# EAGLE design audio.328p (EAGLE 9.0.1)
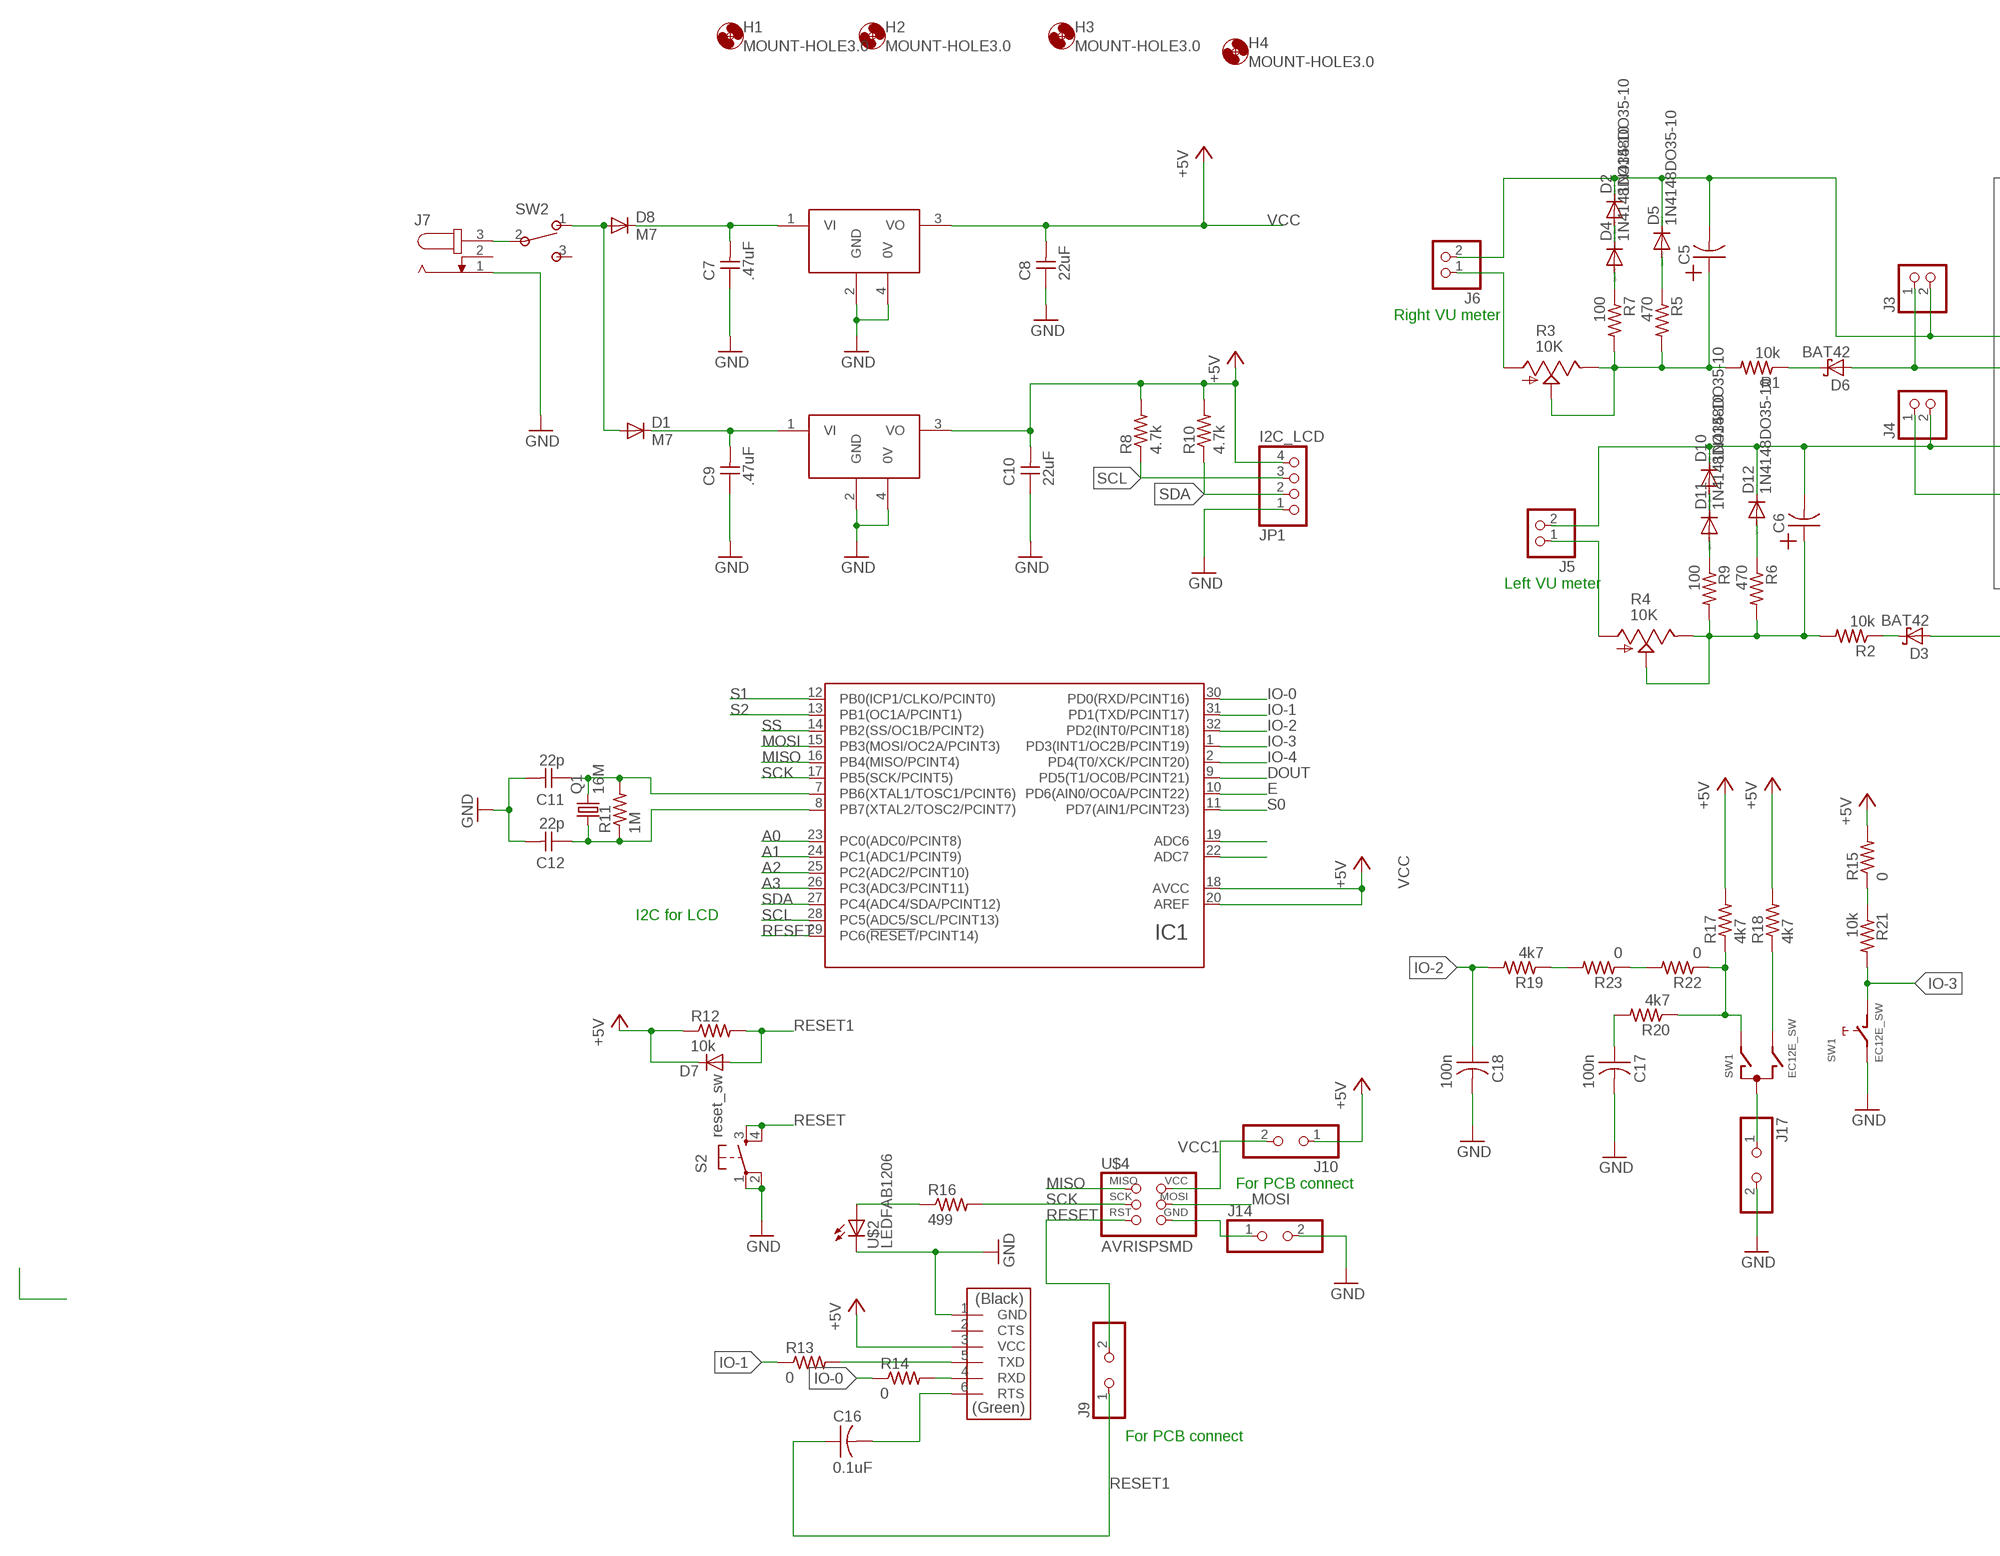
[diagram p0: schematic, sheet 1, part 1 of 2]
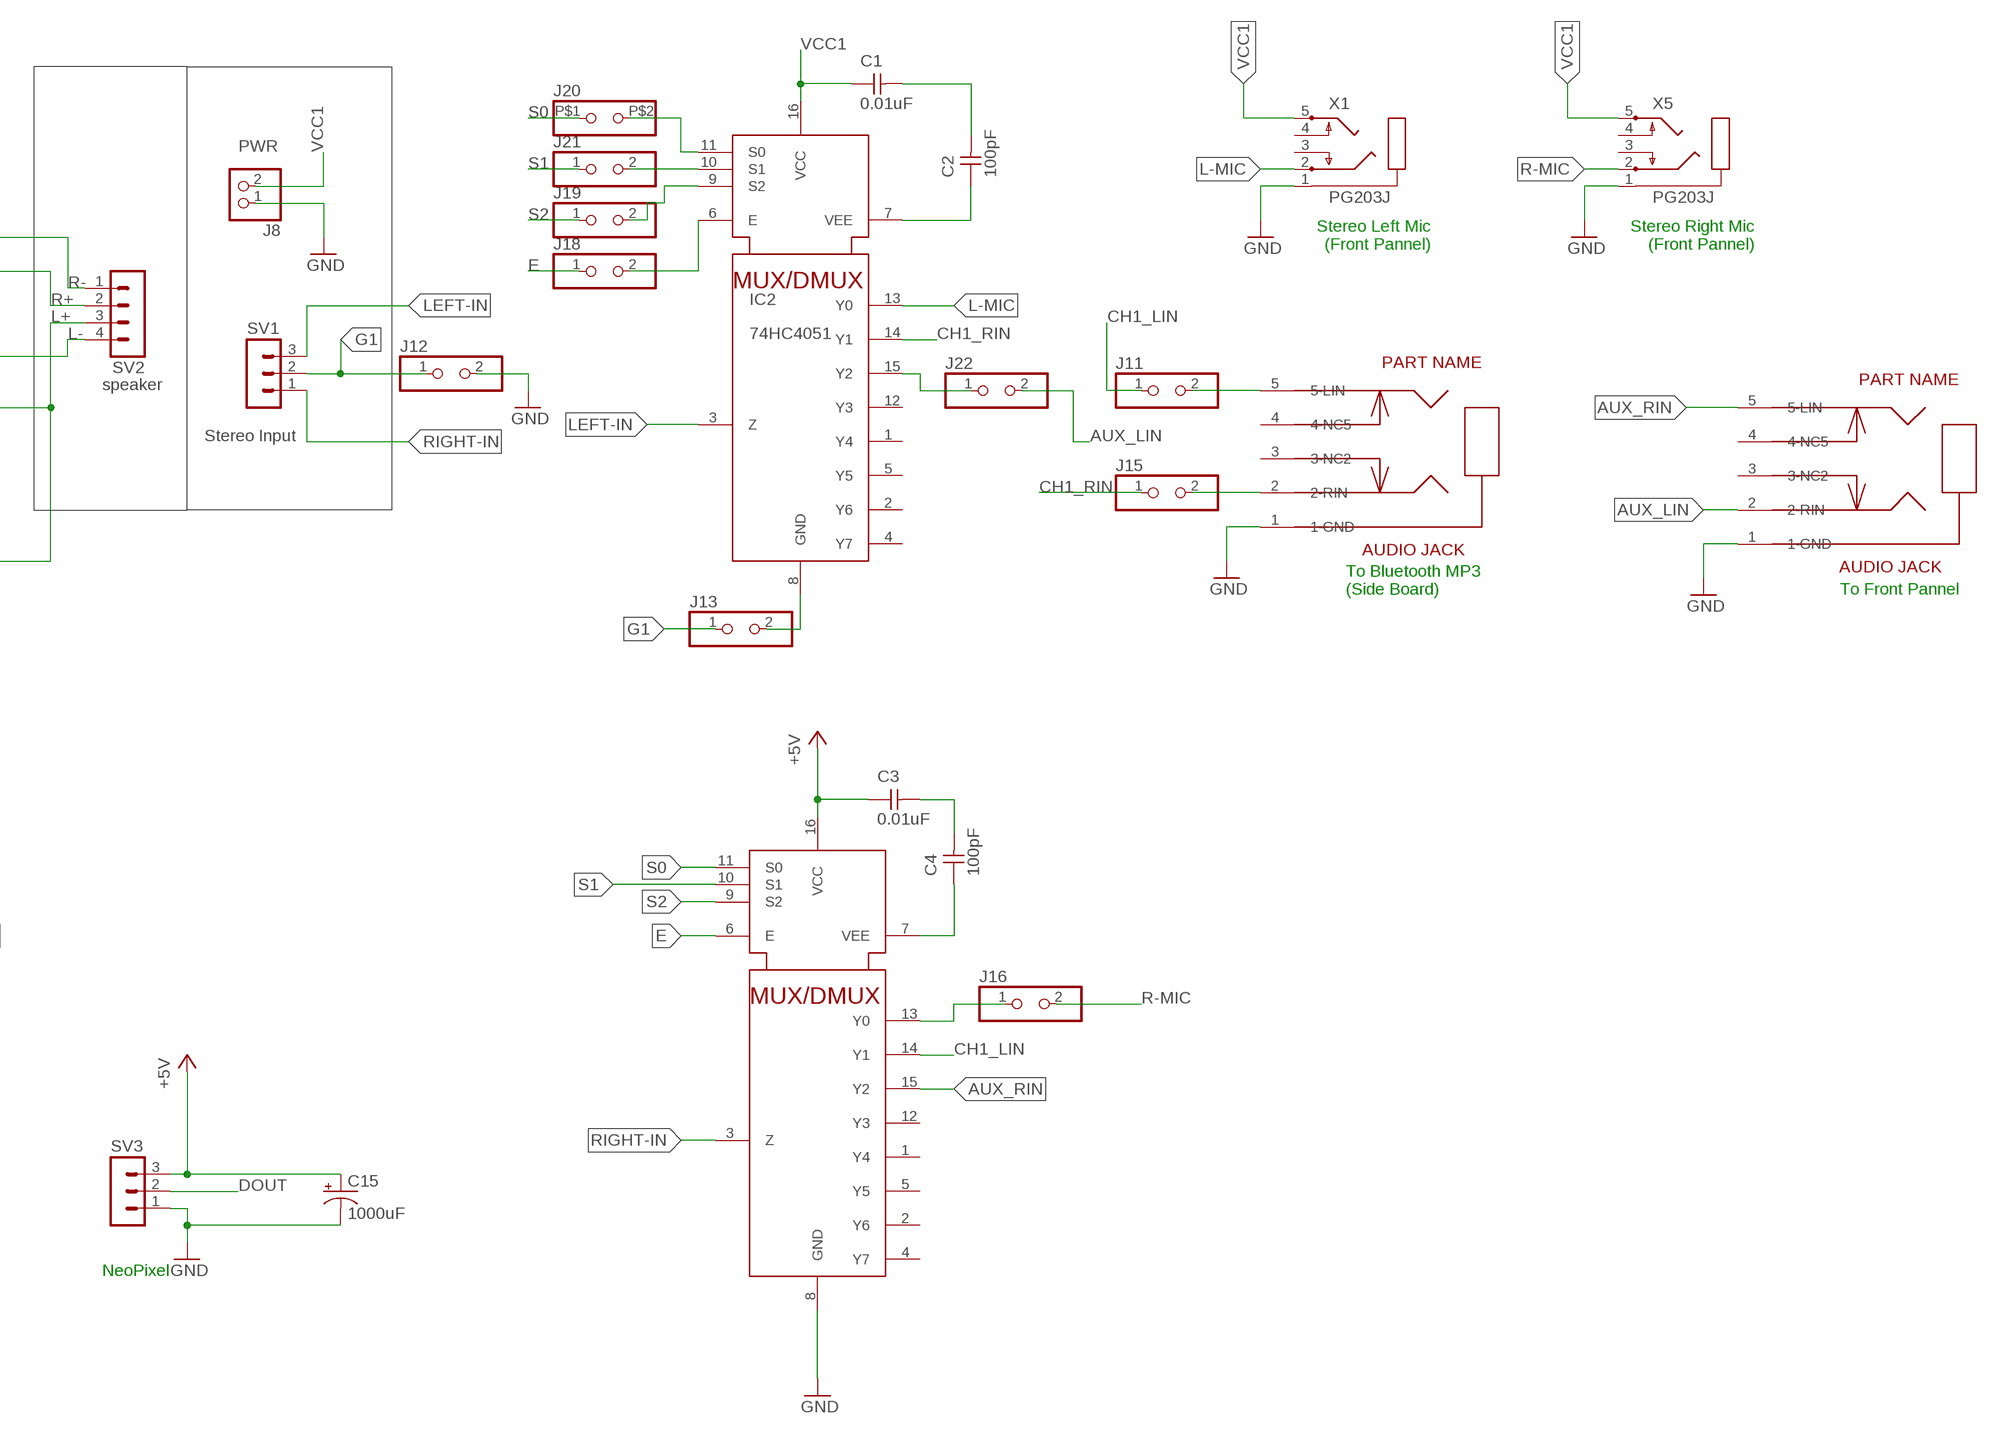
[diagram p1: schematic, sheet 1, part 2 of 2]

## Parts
C1  0.01uF  CAP-UNPOLARIZEDFAB  [C1206FAB]
C2  100pF  CAP-UNPOLARIZEDFAB  [C1206FAB]
C3  0.01uF  CAP-UNPOLARIZEDFAB  [C1206FAB]
C4  100pF  CAP-UNPOLARIZEDFAB  [C1206FAB]
C5  CAP_POL5MM  [5X11MMCAP]
C6  CAP_POL5MM  [5X11MMCAP]
C7  .47uF  CAP-UNPOLARIZEDFAB  [C1206FAB]
C8  22uF  CAP-UNPOLARIZEDFAB  [C1206FAB]
C9  .47uF  CAP-UNPOLARIZEDFAB  [C1206FAB]
C10  22uF  CAP-UNPOLARIZEDFAB  [C1206FAB]
C11  22p  CAP-UNPOLARIZEDFAB  [C1206FAB]
C12  22p  CAP-UNPOLARIZEDFAB  [C1206FAB]
C15  1000uF  CPOL-USE5-10.5  [E5-10,5]
C16  0.1uF  CAP-US1206FAB  [C1206FAB]
C17  100n  CAP-US1206FAB  [C1206FAB]
C18  100n  CAP-US1206FAB  [C1206FAB]
D1  M7  DIODESOD123  [SOD123]
D2  1N4148DO35-10  [DO35-10]
D3  BAT42  [DO35-10]
D4  1N4148DO35-10  [DO35-10]
D5  1N4148DO35-10  [DO35-10]
D6  BAT42  [DO35-10]
D7  DIODESOD123  [SOD123]
D8  M7  DIODESOD123  [SOD123]
D10  1N4148DO35-10  [DO35-10]
D11  1N4148DO35-10  [DO35-10]
D12  1N4148DO35-10  [DO35-10]
H1  MOUNT-HOLE3.0  [3,0]
H2  MOUNT-HOLE3.0  [3,0]
H3  MOUNT-HOLE3.0  [3,0]
H4  MOUNT-HOLE3.0  [3,0]
IC1  ATMEGA48/88/168/328-AU  [TQFP32-08]
IC2  74HC4051  [D_R-PDSO-G16]
IC3  74HC4051  [D_R-PDSO-G16]
J1  BLUE TOOTH  PJ307L  [PJ307L]
J2  PJ307L  [PJ307L]
J3  5267-2P  [MOLEX5267-2P]
J4  5267-2P  [MOLEX5267-2P]
J5  5267-2P  [MOLEX5267-2P]
J6  5267-2P  [MOLEX5267-2P]
J7  JACK-PLUG1  [SPC4078]
J8  5267-2P  [MOLEX5267-2P]
J9  JMPPER18MM  [1X2PJMP18MM]
J10  JMPPER18MM  [1X2PJMP18MM]
J11  JMPPER5M8  [1X2PJMP5M8]
J12  JMPPER5M8  [1X2PJMP5M8]
J13  JMPPER5M8  [1X2PJMP5M8]
J14  JMPPER5M8  [1X2PJMP5M8]
J15  JMPPER5M8  [1X2PJMP5M8]
J16  JMPPER5M8  [1X2PJMP5M8]
J17  JMPPER5M8  [1X2PJMP5M8]
J18  JMPPER5M8  [1X2PJMP5M8]
J19  JMPPER5M8  [1X2PJMP5M8]
J20  JMPPER12MM  [1X2PJMP12MM]
J21  JMPPER5M8  [1X2PJMP5M8]
J22  JMPPER5M8  [1X2PJMP5M8]
JP1  I2C_LCD  PINHD-1X4  [1X04]
M1  FTDI-THT-HEADER  [1X06]
Q1  16M  CRYSTALSM49  [SM49]
R1  10k  RES-US1206FAB  [R1206FAB]
R2  10k  RES-US1206FAB  [R1206FAB]
R3  10K  POT1K_ANGLE  [EVUFXK]
R4  10K  POT1K_ANGLE  [EVUFXK]
R5  470  RES-US1206FAB  [R1206FAB]
R6  470  RES-US1206FAB  [R1206FAB]
R7  100  RES-US1206FAB  [R1206FAB]
R8  4.7k  RES-US1206FAB  [R1206FAB]
R9  100  RES-US1206FAB  [R1206FAB]
R10  4.7k  RES-US1206FAB  [R1206FAB]
R11  1M  RES-US1206FAB  [R1206FAB]
R12  10k  RES-US1206FAB  [R1206FAB]
R13  0  RES-US1206FAB  [R1206FAB]
R14  0  RES-US1206FAB  [R1206FAB]
R15  0  RES-US1206FAB  [R1206FAB]
R16  499  RES-US1206FAB  [R1206FAB]
R17  4k7  RES-US1206FAB  [R1206FAB]
R18  4k7  RES-US1206FAB  [R1206FAB]
R19  4k7  RES-US1206FAB  [R1206FAB]
R20  4k7  RES-US1206FAB  [R1206FAB]
R21  10k  RES-US1206FAB  [R1206FAB]
R22  0  RES-US1206FAB  [R1206FAB]
R23  0  RES-US1206FAB  [R1206FAB]
S2  reset_sw  6MM_SWITCH6MM_SWITCH  [6MM_SWITCH]
SV1  MA03-1  [MA03-1]
SV2  MA04-1  [MA04-1]
SV3  MA03-1  [MA03-1]
SW1  EC12E_SW  [ALPS_EC12E_SW]
SW2  SLIDE-3PSW  [3P5_08]
U1  LM2940-5  LM2940  [SOT223]
U2  LM2940  [SOT223]
U$2  LEDFAB1206  [LED1206FAB]
U$4  AVRISPSMD  [2X03SMD]
X1  PG203J  [PG203J]
X5  PG203J  [PG203J]

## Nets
+5V: C3.1 C10.2 C15.+ D7.CATHODE(C) IC3.16(VCC) J10.1 JP1.4 M1.3(VCC) R8.2 R10.2 R12.1 R15.2 R17.2 R18.2 SV3.3 U2.3(VO)
A0: IC1.23(PC0(ADC0/PCINT8))
A1: IC1.24(PC1(ADC1/PCINT9))
A2: IC1.25(PC2(ADC2/PCINT10))
A3: IC1.26(PC3(ADC3/PCINT11))
AUX_LIN: J2.2(2-RIN) J22.2
AUX_RIN: IC3.15(Y2) J2.5(5-LIN)
CH1_LIN: IC3.14(Y1) J11.1
CH1_RIN: IC2.14(Y1) J15.1
DOUT: IC1.9(PD5(T1/OC0B/PCINT21)) SV3.2
E: IC1.10(PD6(AIN0/OC0A/PCINT22)) IC3.6(E) J18.1
G1: J12.1 J13.1 SV1.2
GND: C7.1 C8.1 C9.1 C10.1 C11.2 C12.2 C15.- C17.2 C18.2 IC3.8(GND) J1.1(1-GND) J2.1(1-GND) J7.1 J8.1 J12.2 J14.2 J17.2 JP1.1 M1.1(GND) S2.1(P) S2.2(P1) SV3.1 SW1.E U1.2(GND) U1.4(0V) U2.2(GND) U2.4(0V) U$2.2(C) X1.1 X5.1
IO-0: IC1.30(PD0(RXD/PCINT16)) R14.1
IO-1: IC1.31(PD1(TXD/PCINT17)) R13.1
IO-2: C18.1 IC1.32(PD2(INT0/PCINT18)) R19.2
IO-3: IC1.1(PD3(INT1/OC2B/PCINT19)) R21.2 SW1.D
IO-4: IC1.2(PD4(T0/XCK/PCINT20))
L+: D3.A J4.1 SV2.3
L-: C6.P$2(M) D10.C D12.C J4.2 J5.2 SV2.4
L-MIC: IC2.13(Y0) X1.2
LEFT-IN: IC2.3(Z) SV1.3
MISO: IC1.16(PB4(MISO/PCINT4)) U$4.1(MISO)
MOSI: IC1.15(PB3(MOSI/OC2A/PCINT3)) U$4.4(MOSI)
N$1: C1.2 C2.2
N$2: C2.1 IC2.7(VEE)
N$3: C3.2 C4.2
N$4: C4.1 IC3.7(VEE)
N$5: J7.3 SW2.2
N$6: C7.2 D8.CATHODE(C) U1.1(VI)
N$8: IC1.19(ADC6)
N$9: D11.A R9.1
N$10: D12.A R6.1
N$11: D10.A D11.C
N$12: D6.C R1.1
N$13: C6.P$1(P) R2.2 R4.2(S) R4.3(E) R6.2 R9.2
N$14: J5.1 R4.1(A)
N$15: C9.2 D1.CATHODE(C) U2.1(VI)
N$16: C5.P$1(P) R1.2 R3.2(S) R3.3(E) R5.2 R7.2
N$18: D4.A R7.1
N$19: D5.A R5.1
N$20: D2.A D4.C
N$21: J6.1 R3.1(A)
N$22: IC1.22(ADC7)
N$26: C11.1 IC1.7(PB6(XTAL1/TOSC1/PCINT6)) Q1.2 R11.2
N$27: C12.1 IC1.8(PB7(XTAL2/TOSC2/PCINT7)) Q1.1 R11.1
N$28: R16.1 U$2.1(A)
N$29: R18.1 SW1.B
N$30: C16.2 M1.6(RTS)
N$31: R17.1 R20.1 R22.1 SW1.A
N$32: C17.1 R20.2
N$33: D1.ANODE(A) D8.ANODE(A) SW2.1
N$34: M1.4(RXD) R14.2
N$35: M1.5(TXD) R13.2
N$36: R15.1 R21.1
N$37: R19.1 R23.2
N$38: R22.2 R23.1
N$39: J1.2(2-RIN) J15.2
N$40: J14.1 U$4.6(GND)
N$41: IC2.8(GND) J13.2
N$42: J1.5(5-LIN) J11.2
N$43: J17.1 SW1.C
N$44: IC3.13(Y0) J16.1
N$45: IC2.10(S1) J21.2
N$46: IC2.11(S0) J20.P$2
N$47: IC2.9(S2) J19.2
N$48: IC2.6(E) J18.2
N$49: IC2.15(Y2) J22.1
N$50: D3.C R2.1
R+: D6.A J3.1 SV2.2
R-: C5.P$2(M) D2.C D5.C J3.2 J6.2 SV2.1
R-MIC: J16.2 X5.2
RESET: IC1.29(PC6(!RESET!/PCINT14)) J9.2 S2.3(S) S2.4(S1) U$4.5(RST)
RESET1: C16.1 D7.ANODE(A) J9.1 R12.2
RIGHT-IN: IC3.3(Z) SV1.1
S0: IC1.11(PD7(AIN1/PCINT23)) IC3.11(S0) J20.P$1
S1: IC1.12(PB0(ICP1/CLKO/PCINT0)) IC3.10(S1) J21.1
S2: IC1.13(PB1(OC1A/PCINT1)) IC3.9(S2) J19.1
SCK: IC1.17(PB5(SCK/PCINT5)) R16.2 U$4.3(SCK)
SCL: IC1.28(PC5(ADC5/SCL/PCINT13)) JP1.3 R8.1
SDA: IC1.27(PC4(ADC4/SDA/PCINT12)) JP1.2 R10.1
SS: IC1.14(PB2(SS/OC1B/PCINT2))
VCC: C8.2 IC1.18(AVCC) IC1.20(AREF) U1.3(VO) ; supply symbol labelled +5V
VCC1: C1.1 IC2.16(VCC) J8.2 J10.2 U$4.2(VCC) X1.5 X5.5
Unconnected: IC2.1(Y4) IC2.2(Y6) IC2.4(Y7) IC2.5(Y5) IC2.12(Y3) IC3.1(Y4) IC3.2(Y6) IC3.4(Y7) IC3.5(Y5) IC3.12(Y3) J1.3(3-NC2) J1.4(4-NC5) J2.3(3-NC2) J2.4(4-NC5) J7.2 M1.2(CTS) SW1.GND1(G) SW1.GND2(G) SW2.3 X1.3 X1.4 X5.3 X5.4

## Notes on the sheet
- PWR
- Right VU meter
- Stereo Left Mic
  (Front Pannel)
- Stereo Right Mic
  (Front Pannel)
- speaker
- Stereo Input
- Left VU meter
- To Bluetooth MP3
  (Side Board)
- To Front Pannel
- I2C for LCD
- For PCB connect
- NeoPixel
- For PCB connect

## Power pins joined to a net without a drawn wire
GND: IC1.3(GND) IC1.5(GND) IC1.21(GND)
VCC: IC1.4(VCC) IC1.6(VCC)

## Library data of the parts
C1-C4 C7-C12 = fab:CAP-UNPOLARIZED
C5 C6 = discrete_ys:CAP_POL5MM
C15 = rcl:CPOL-US: POLARIZED CAPACITOR, American symbol; SPICEPREFIX: C
C16-C18 = fab:CAP-US
D1 D7 D8 = fab:DIODE: DIODE
D2 D4 D5 D10-D12 = diode:1N4148: DIODE
D3 D6 = diode:BAT42: DIODE
H1-H4 = holes:MOUNT-HOLE: MOUNTING HOLE with drill center marker
IC1 = atmel_tiny24-44-84tiny48-88mega48-88-168-328:ATMEGA48/88/168/328
IC2 IC3 = audio_basic:74HC4051
J1 J2 = audio_basic:PJ307L
J3-J6 J8 = connector_ys:5267-2P
J7 = con-jack:JACK-PLUG: DC POWER JACK Power Jack, DC, Right Angle, Through Hole, Rated 5A at 16VDC, PC Terminals Distributor: Farnell (www.Farnell.de) Drawing: 84N1161.pdf / 84N1162.pdf Manufacturer: SPC Technology (www.spctechnology.com) Type: SPC4077 / SPC 4078; OC_FARNELL: unknown; OC_NEWARK: unknown
J9 J10 = discrete_ys:JMPPER18MM
J11-J19 J21 J22 = discrete_ys:JMPPER5M8
J20 = discrete_ys:JMPPER12MM
JP1 = pinhead:PINHD-1X4: PIN HEADER
M1 = fab:FTDI-THT-HEADER
Q1 = crystal:CRYSTAL: CRYSTAL; OC_FARNELL: unknown; OC_NEWARK: unknown
R1 R2 R5-R23 = fab:RES-US: Resistor (US Symbol)
R3 R4 = discrete_ys:POT1K_ANGLE
S2 = fab:6MM_SWITCH: OMRON SWITCH
SV1 SV3 = con-lstb:MA03-1: PIN HEADER; OC_FARNELL: unknown; OC_NEWARK: unknown
SV2 = con-lstb:MA04-1: PIN HEADER; OC_FARNELL: unknown; OC_NEWARK: unknown
SW1 = switch-alps:EC12E_SW: ALPS rotary Encoder EC12E series with switch; MPN: EC12E2424407; OC_FARNELL: 1520813; OC_NEWARK: 74M1068
SW2 = connector_ys:SLIDE-3PSW
U1 U2 = discrete_ys:LM2940
U$2 = fab:LED: LED
U$4 = fab:AVRISP
X1 X5 = con-hirschmann:PG203J: MIC/HEADPHONE JACK KS-S stereo microphone/headphone jack PG203JN (Schukat); OC_FARNELL: unknown; OC_NEWARK: unknown

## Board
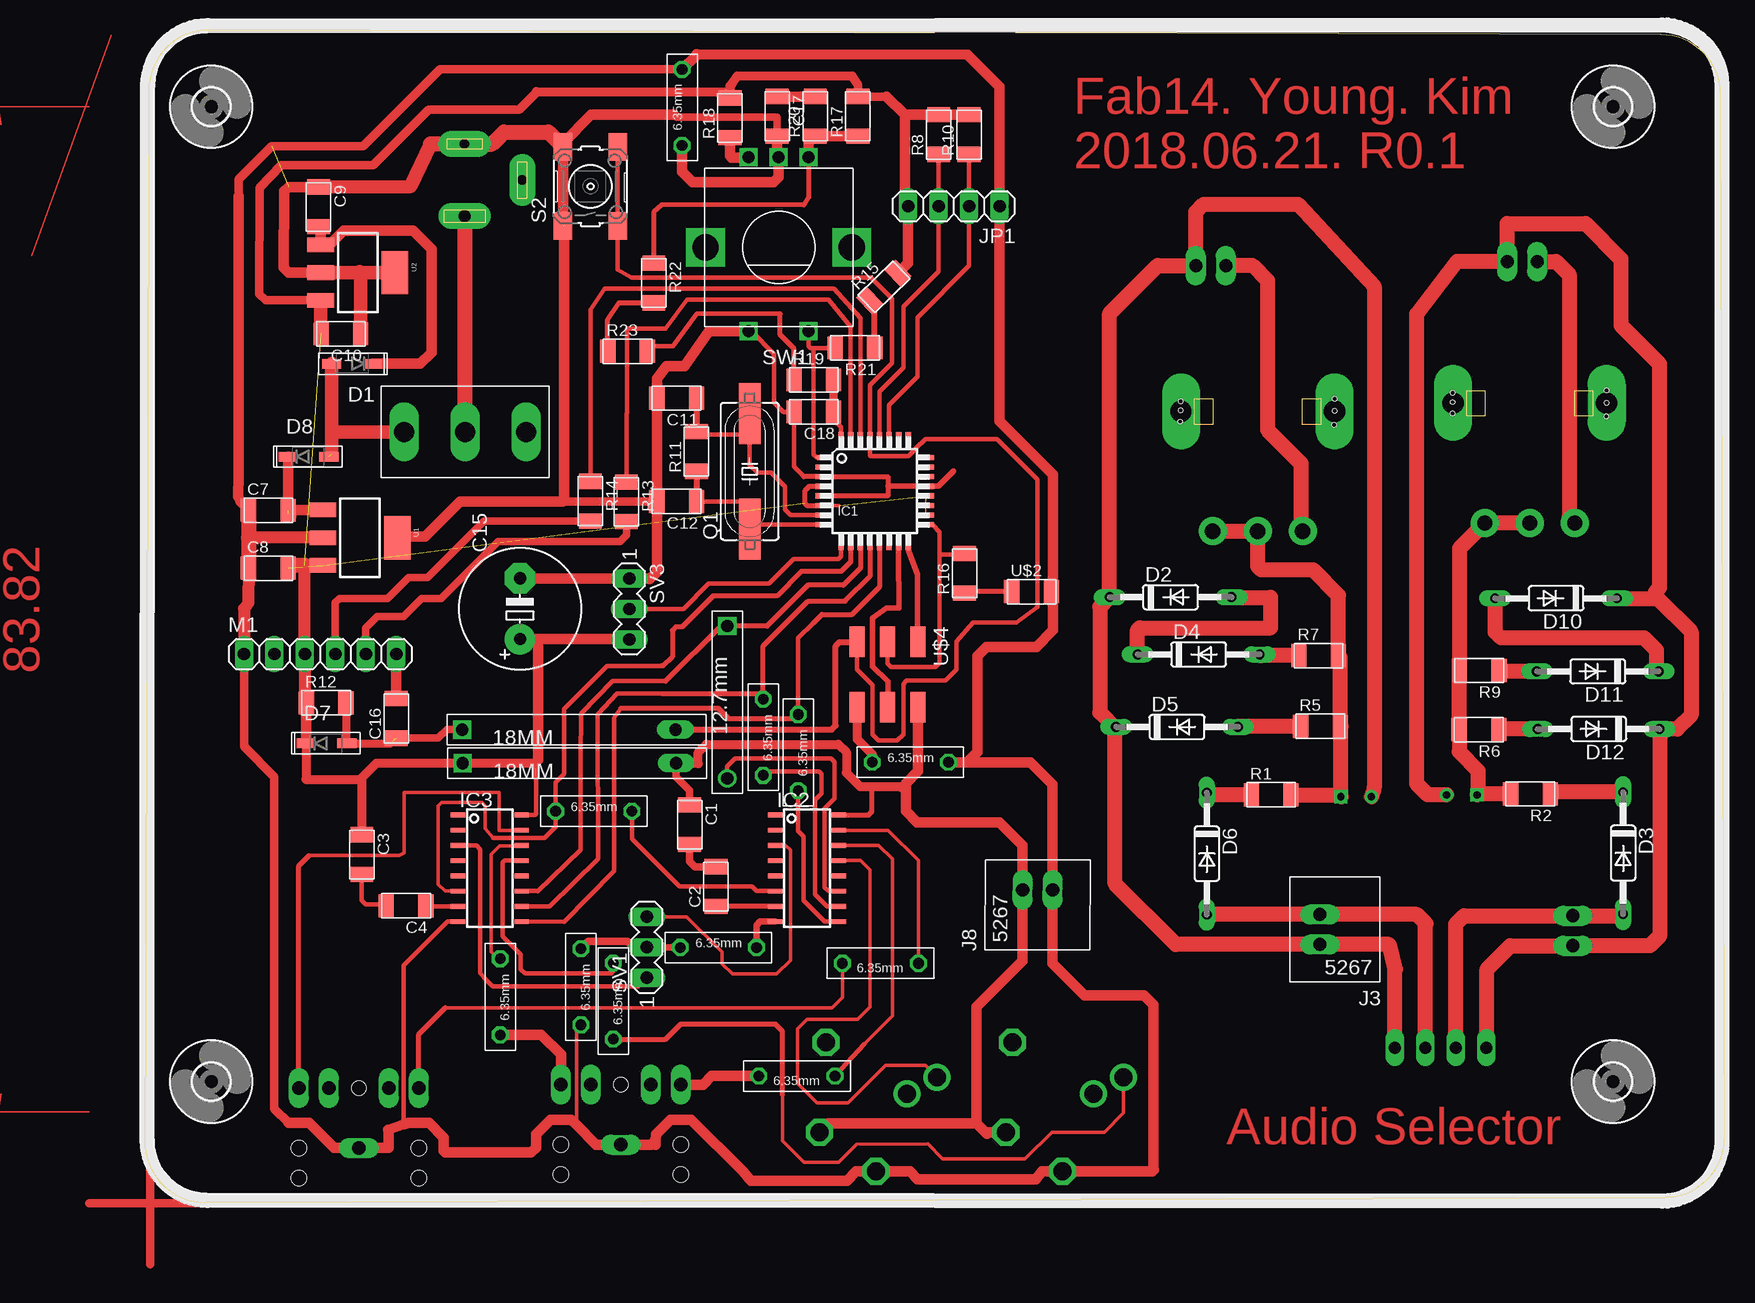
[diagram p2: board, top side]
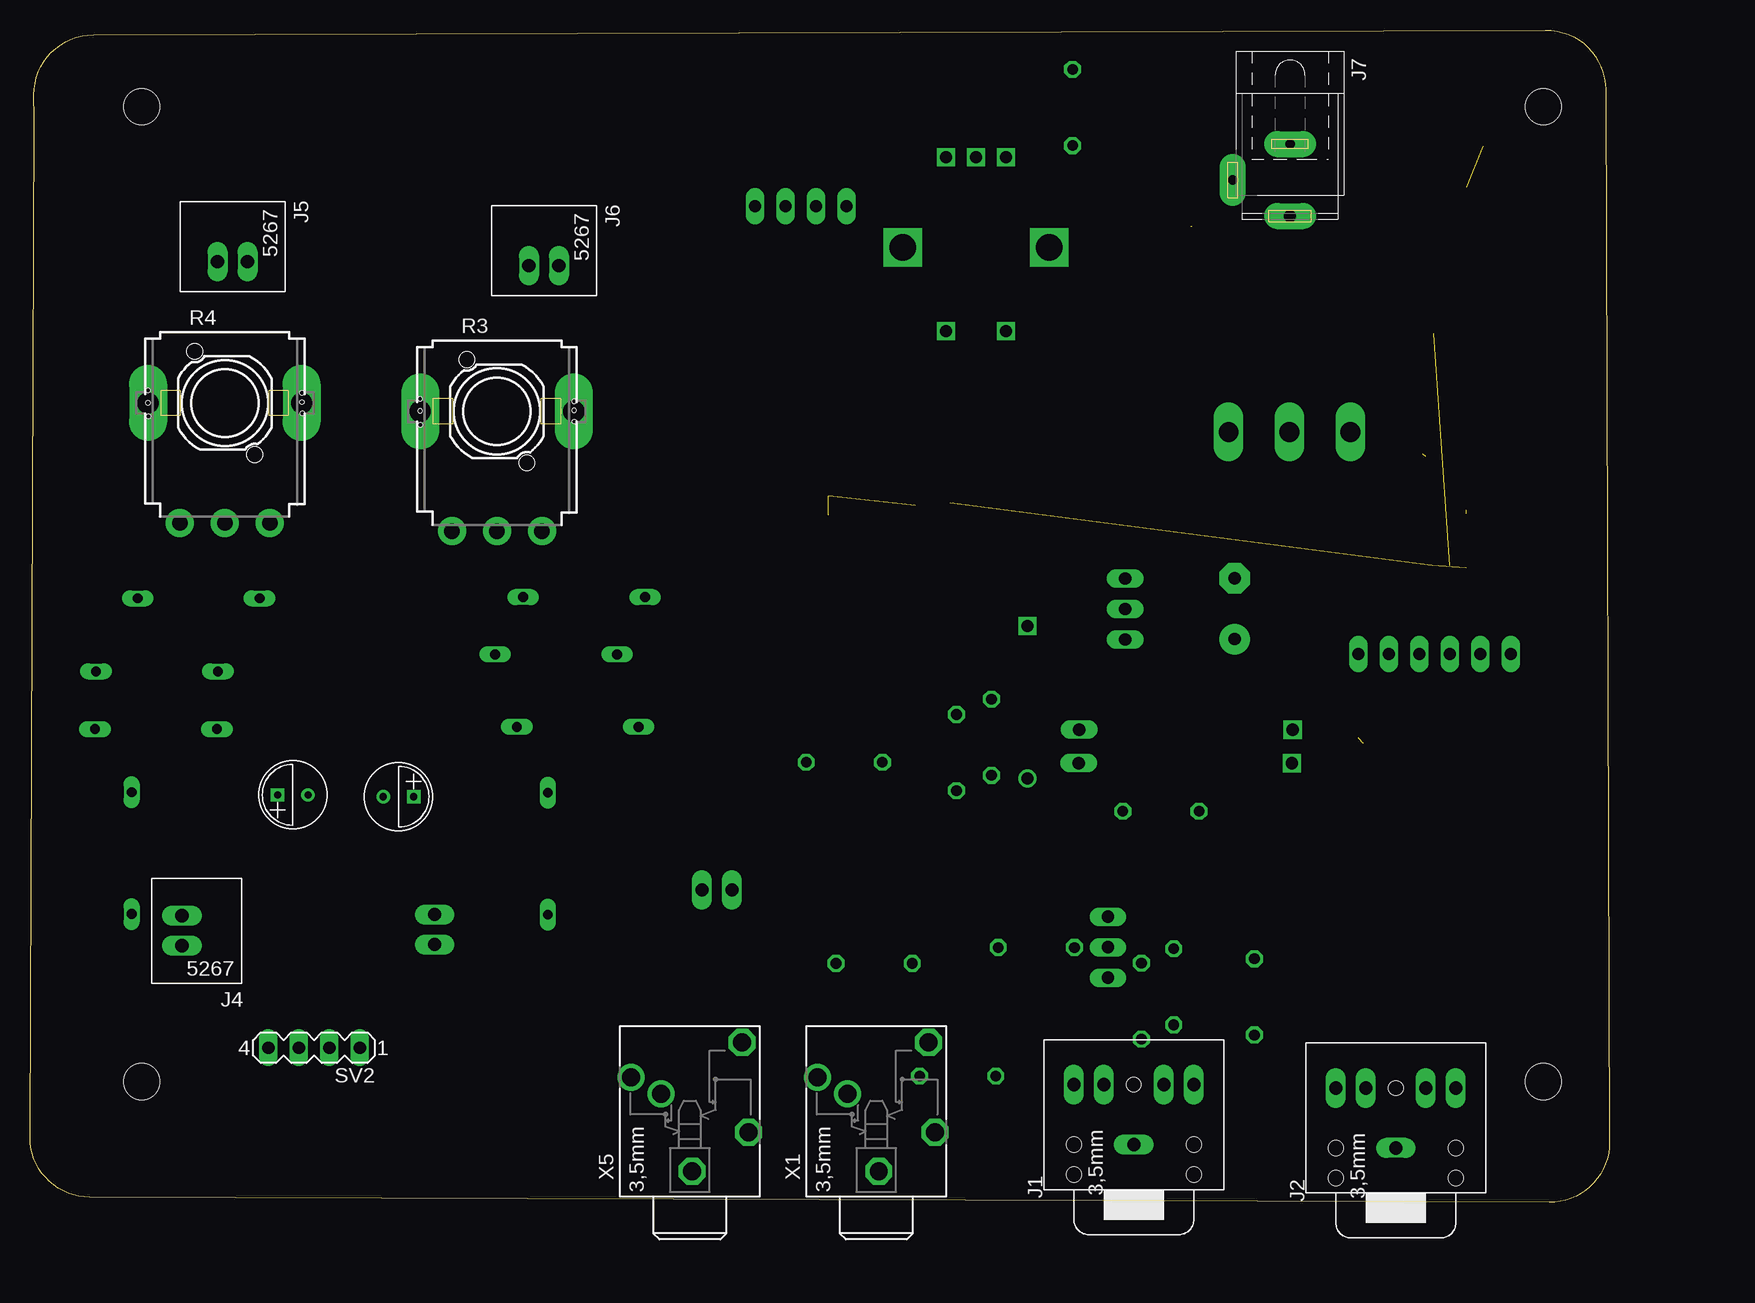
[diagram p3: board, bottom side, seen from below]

Size 131.67 x 97.73 mm. Coordinates in mm from the lower left corner, seen from the top.
Outline: 131.33,90.36 131.34,92.32 arc90 126.35,97.33 5.34,97.73 arc90 0.32,92.75 0,5.02 arc90 5.02,0 126.68,0.42 arc90 131.67,5.44 131.33,90.36
Copper layers (1*16): Top 0.035mm / dielectric 1.5mm / Bottom 0.035mm
Design rules "default *": minimum track width 6mil, minimum drill 0.35mm, track to track 6mil, track to pad 1mil, pad to pad 6mil, via to via 6mil, smd to smd 6mil, copper to edge 40mil, drill to drill 6mil, minimum pad ring 10mil, minimum via ring 8mil, stop-mask expansion 4mil, vias tented up to drill 0mil, thermal gap 10mil

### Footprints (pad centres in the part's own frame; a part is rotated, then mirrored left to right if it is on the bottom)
C1206FAB = smd 1.27 x 1.905: 1 -1.651,0; 2 1.651,0
5X11MMCAP = drill 0.6 square: P$1 0,1.27 | drill 0.6: P$2 0,-1.27
E5-10,5 = drill 1.016 pad 2.54: + -2.54,0 | drill 1.016 pad 2.54 octagon: - 2.54,0
SOD123 = smd 1.6 x 0.8: ANODE 1.7,0; CATHODE -1.7,0
DO35-10 = drill 0.813 long: A 5.08,0; C -5.08,0
3,0 = hole 3: 0,0
TQFP32-08 = smd 1.27 x 0.457: 1 -4.293,2.8 | smd 1.27 x 0.432: 2 -4.293,2; 3 -4.293,1.2; 4 -4.293,0.4; 5 -4.293,-0.4; 6 -4.293,-1.2; 7 -4.293,-2; 8 -4.293,-2.8; 17 4.293,-2.8; 18 4.293,-2; 19 4.293,-1.2; 20 4.293,-0.4; 21 4.293,0.4; 22 4.293,1.2; 23 4.293,2; 24 4.293,2.8 | smd 0.432 x 1.27: 9 -2.8,-4.293; 10 -2,-4.293; 11 -1.2,-4.293; 12 -0.4,-4.293; 13 0.4,-4.293; 14 1.2,-4.293; 15 2,-4.293; 16 2.8,-4.293; 25 2.8,4.293; 26 2,4.293; 27 1.2,4.293; 28 0.4,4.293; 29 -0.4,4.293; 30 -1.2,4.293; 31 -2,4.293; 32 -2.8,4.293
D_R-PDSO-G16 = smd 0.4 x 1.2: 1 -4.445,-2.65; 2 -3.175,-2.65; 3 -1.905,-2.65; 4 -0.635,-2.65; 5 0.635,-2.65; 6 1.905,-2.65; 7 3.175,-2.65; 8 4.445,-2.65; 9 4.445,2.65; 10 3.175,2.65; 11 1.905,2.65; 12 0.635,2.65; 13 -0.635,2.65; 14 -1.905,2.65; 15 -3.175,2.65; 16 -4.445,2.65
PJ307L = drill 1.1 long: 1 0,0; 2 5,5; 3 5,2.5; 4 5,-2.5; 5 5,-5 | hole 1.2: 5,0 | hole 1.25: 0,-5; -2.5,-5; 0,5; -2.5,5
MOLEX5267-2P = drill 1.1 long: 1 -1.25,-1.25; 2 -1.25,1.25
SPC4078 = drill 0.8 pad 2.184 long: 1 -3,0; 2 0,-4.8 | drill 1 pad 2.184 long: 3 3,0
1X2PJMP18MM = drill 1.016 square: 1 0,0 | drill 1.016 long: 2 17.78,0
1X2PJMP5M8 = drill 0.889 octagon: 1 0,0; 2 6.35,0
1X2PJMP12MM = drill 1.016 square: P$1 0,0 | drill 1.016: P$2 12.7,0
1X04 = drill 1.016 long: 1 -3.81,0; 2 -1.27,0; 3 1.27,0; 4 3.81,0
1X06 = drill 1.016 long: 1 -6.35,0; 2 -3.81,0; 3 -1.27,0; 4 1.27,0; 5 3.81,0; 6 6.35,0
SM49 = smd 5.08 x 1.778: 1 -4.826,0; 2 4.826,0
R1206FAB = smd 1.27 x 1.905: 1 -1.651,0; 2 1.651,0
EVUFXK = drill 1.27 pad 2.337: 1 -3.75,-10; 2 0,-10; 3 3.75,-10 | drill 1.778 pad 3.175 long: M1 6.4,0; M2 -6.4,0 | hole 0.35: 6.426,0.838; 6.426,0.076; 6.452,-0.864; -6.401,1.041; -6.401,0.025; -6.375,-1.118
6MM_SWITCH = smd 2.286 x 1.524: 1 -3.302,2.286; 2 3.302,2.286; 3 -3.302,-2.286; 4 3.302,-2.286
MA03-1 = drill 1.016 long: 1 -2.54,0; 2 0,0; 3 2.54,0
MA04-1 = drill 1.016 long: 1 -3.81,0; 2 -1.27,0; 3 1.27,0; 4 3.81,0
ALPS_EC12E_SW = drill 1 square: A -2.5,-7.5; B 2.5,-7.5; C 0,-7.5; D -2.5,7; E 2.5,7 | drill 2.2 square: GND1 -6.1,0; GND2 6.1,0
3P5_08 = drill 1.651 long: 1 0,5.08; 2 0,0; 3 0,-5.08
SOT223 = smd 1.219 x 2.235: 1 -2.311,-3.099; 2 0,-3.099; 3 2.311,-3.099 | smd 3.6 x 2.2: 4 0,3.099
LED1206FAB = smd 1.27 x 1.905: 1 -1.651,0; 2 1.651,0
2X03SMD = smd 2.54 x 1.27: 1 -2.54,2.54; 2 2.92,2.54; 3 -2.54,0; 4 2.92,0; 5 -2.54,-2.54; 6 2.92,-2.54
PG203J = drill 1.499 octagon: 1 -5.004,-0.203; 4 5.74,-4.369; 5 -1.753,-4.902 | drill 1.499: 2 2.845,4.902; 3 1.448,2.388

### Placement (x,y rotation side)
C1  45.4,31.48 270 top
C2  47.58,26.32 90 top
C3  18.07,28.99 270 top
C4  21.75,24.72 180 top
C5  100.95,33.82 270 bottom
C6  109.76,33.97 90 bottom
C7  10.27,57.69 0 top
C8  10.27,52.87 0 top
C9  14.46,82.99 270 top
C10  16.31,72.4 180 top
C11  44.3,67.04 180 top
C12  44.3,58.43 180 top
C15  31.25,49.49 90 top
C16  20.94,40.34 90 top
C17  52.69,90.53 270 top
C18  55.73,65.9 180 top
D1  17.25,69.91 180 top
D2  85.48,50.45 0 top
D3  123.2,29.12 270 top
D4  87.81,45.68 0 top
D5  86.01,39.63 0 top
D6  88.5,29.07 270 top
D7  15.12,38.26 0 top
D8  13.62,62.16 0 top
D10  117.61,50.35 180 top
D11  121.09,44.25 180 top
D12  121.16,39.45 180 top
H1  122.36,10.07 0 top
H2  5.52,10.07 0 top
H3  122.36,91.35 0 top
H4  5.52,91.35 0 top
IC1  60.81,59.29 0 top
IC2  55.18,27.85 270 top
IC3  28.73,27.85 270 top
J1  39.66,4.81 90 bottom
J2  17.81,4.53 90 bottom
J3  96.68,22.74 180 top
J4  120.25,22.64 180 bottom
J5  114.79,77.17 270 bottom
J6  88.83,76.84 270 bottom
J7  26.63,85.22 270 bottom
J8  74.4,27.29 89.9 top
J9  26.42,39.4 0 top
J10  26.47,36.61 0 top
J11  29.6,20.3 270 top
J12  36.33,21.14 270 top
J13  44.61,21.24 0 top
J14  60.61,36.69 0 top
J15  57.51,10.52 180 top
J16  39.02,19.95 270 top
J17  44.76,88.1 90 top
J18  34.22,32.6 0 top
J19  54.44,40.67 270 top
J20  48.52,48.04 270 top
J21  51.52,41.94 270 top
J22  64.47,19.92 180 top
JP1  67.42,83.04 180 top
M1  14.59,45.7 0 top
Q1  50.4,60.94 90 top
R1  93.86,33.97 0 top
R2  115.48,34.04 180 top
R3  92.74,65.95 0 bottom
R4  115.42,66.63 0 bottom
R5  97.97,39.68 0 top
R6  111.18,39.4 180 top
R7  97.82,45.58 0 top
R8  66.15,89.01 90 top
R9  111.21,44.33 180 top
R10  68.69,89.01 90 top
R11  45.96,62.59 90 top
R12  15.09,41.64 0 top
R13  40.11,58.4 270 top
R14  37.12,58.45 270 top
R15  61.58,76.31 44.1 top
R16  68.31,52.43 90 top
R17  59.42,90.53 90 top
R18  48.75,90.41 90 top
R19  55.73,68.56 0 top
R20  55.86,90.53 90 top
R21  59.16,71.23 180 top
R22  42.4,76.64 270 top
R23  40.22,70.95 0 top
S2  37.12,84.69 90 top
SV1  41.82,21.27 90 top
SV2  107.98,12.89 180 bottom
SV3  40.37,49.46 270 top
SW1  52.81,79.61 180 top
SW2  26.68,64.22 90 top
U1  17.91,55.41 270 top
U2  17.74,77.5 270 top
U$2  73.9,50.91 0 top
U$4  61.88,44.18 270 top
X1  61.12,7.58 90 bottom
X5  76.66,7.58 90 bottom

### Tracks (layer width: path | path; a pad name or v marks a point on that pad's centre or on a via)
+5V  (1 unrouted)
  Top 0.356: IC3.16 32.49,32.29 32.57,32.37 32.57,36.69
  Top 0.711: U2.3 10.04,75.19 9.51,75.73 9.53,84.56 11.34,86.44 19.01,86.44 23.63,91.07 31.17,91.07 32.59,92.49 32.59,92.59 | 61.8,92.18 R17.2 59.42,93.18 58.93,93.89 | R18.2 48.24,92.57
  Top 0.762: 32.59,92.59 48.24,92.57 | 58.93,93.89 49.36,93.89 48.9,93.2 48.75,93.05 R18.2 | D7.CATHODE 13.42,35.26 13.44,35.24 17.91,35.24 | 17.91,35.24 18.07,35.09 C3.1 | 17.91,35.24 19.29,36.61 J10.1 32.49,36.61 32.57,36.69 32.77,36.89
  Top 0.889: R12.1 13.44,38.69 D7.CATHODE | R10.2 R8.2 63.33,90.66 | 61.8,92.18 63.33,90.66 | 63.33,90.66 63.33,83.32 JP1.4 63.61,78.31 R15.2 | C15.+ 32.65,46.95 | 32.65,46.95 40.34,46.95 SV3.3 | 32.77,36.89 32.77,46.82 32.65,46.95
  Top 1.016: 13.32,53.09 M1.3 13.32,41.77 R12.1
  Top 1.143: U2.3 14.64,72.42 C10.2
  Top 1.27: 13.32,53.09 12.15,53.09
AUX_LIN
  Top 0.305: J22.2 58.12,17.08 57.26,16.21 25.03,16.21
  Top 0.406: J2.2 22.81,14 25.03,16.21
AUX_RIN
  Top 0.305: IC3.15 29.5,31.02 29.5,34.17 21.6,34.17 21.6,29.12 21.19,28.91 13.67,28.91
  Top 0.406: J2.5 12.81,28.05 13.67,28.91
CH1_LIN
  Top 0.305: IC3.14 arc-90 31.36,29.73 29.55,29.73 28.84,29.01 28.84,20.86 29.39,20.3 J11.1
CH1_RIN
  Top 0.305: 59.98,13.22 62.29,15.53 62.29,28.61 61.14,29.75 IC2.14
  Top 0.356: J15.1 59.98,13.22
DOUT
  Top 0.356: IC1.9 58.01,53.85 57.79,53.63 54.06,53.63 52,51.57 46.97,51.57 44.86,49.46 SV3.2
E
  Top 0.305: IC3.6 25,25.94 24.44,26.5 24.44,33.05 24.72,33.33 28.07,33.33 28.35,33.05 28.35,31.16 29.02,30.39
  Top 0.356: 43.01,44.71 38.49,44.71 34.91,41.13 34.91,35.7 34.22,35.01 J18.1 34.22,31.3 33.31,30.39 29.02,30.39
  Top 0.406: IC1.10 58.81,53.38 58.02,52.59 54.69,52.59 52.66,50.55 47.35,50.55 44.76,47.96 44.23,47.96 43.95,47.68 43.95,45.47 43.19,44.71 43.01,44.71
G1
  Top 0.559: J13.1 41.84,21.24 SV1.2
  Top 0.61: SV1.2 40.7,21.27 40.21,21.75 36.94,21.75 J12.1
GND  (2 unrouted)
  Top 0.305: 35.96,14.3 35.96,14.28 35.96,6.45
  Top 0.356: IC3.8 25.2,23.4 21.56,19.76 21.56,6.49 | J12.2 35.96,14.43 35.96,14.28
  Top 0.381: 54.92,60.49 54.08,61.32 C18.2 53.19,65.9 52.43,66.66 52.43,70.72 50.54,72.61 SW1.E
  Top 0.406: IC1.5 57.87,58.89 61.91,58.89 61.91,59.72 61.91,60.49 57.96,60.49 IC1.3 54.92,60.49 | U$2.2 75.55,48.81 75.69,48.67
  Top 0.457: 61.91,59.72 62,59.69 IC1.21 66.14,59.69 67.39,60.94
  Top 0.61: C17.2 52.69,90.46 44.28,90.46 44.08,90.66
  Top 0.711: C12.2 34.8,58.43 | J17.2 24.59,94.45 18.19,88.04 10.55,88.04 7.82,85.31 7.82,83.87 | 11.95,6.61 10.75,7.81 10.75,35.47 8.24,37.98 M1.1
  Top 0.889: 34.91,81.39 34.93,75.34 34.93,58.56 34.8,58.43 26.24,58.43 23.32,55.51 21.11,55.51 U1.4 | 44.08,90.66 37.19,90.66 34.78,88.25 34.78,87.95 | 52.69,87.24 C17.2 | SW1.E 46.99,72.61 44.96,69.71 43.47,69.71 42.65,68.66 C11.2 C12.2 42.65,52.56 42.07,51.98 42.04,52 SV3.1 31.27,52 C15.- | U2.2 11.94,77.5 11.54,77.91 11.59,84.31 11.94,84.62 C9.1 | S2.1 S2.2 | 7.82,83.87 7.79,60.69 7.75,58.84 7.98,58.4 8.62,57.77 C7.1 | 11.95,6.61 13.68,6.61 15.76,4.53 J2.1 17.84,4.55 20.3,4.55 20.29,5.89 20.27,6.05 21.56,6.49 21.95,6.61 23.68,6.61 24.9,5.39 24.9,4.3 25.02,4.17 32.19,4.17 32.57,4.56 32.57,5.67 33.79,6.89 35.52,6.89 35.96,6.45 37.61,4.81 J1.1 42.17,4.81 42.55,5.18 | 42.55,5.18 42.57,5.67 43.79,6.89 45.52,6.89 49.84,2.57 50.4,1.94 50.53,1.81 58.5,1.81 59.26,2.57 X1.1 63.76,2.57 64.4,1.94 74.25,1.94 74.3,1.99 74.66,2.47 74.76,2.57 X5.1 83.95,2.57 84.08,2.7 84.03,2.75 84.03,16.47 83.24,17.25 78.31,17.25 75.65,19.92 J8.1 75.65,34.85 73.82,36.69 J14.2 68.51,36.69 69.37,37.55 69.37,45.55 70.12,46.3 74.3,46.3 75.69,47.69 75.69,48.67 75.69,60.68 71.23,65.14 JP1.1 71.23,93 68.56,95.66 45.96,95.69 45.96,95.64 J17.2 | 42.55,5.18 42.55,4.81
  Top 1.016: U1.2 8.62,55.41 | C8.1 8.59,50 8.24,49.46 M1.1
  Top 1.143: U2.4 17.99,77.5 | 17.99,77.5 U2.2 | C10.1 17.96,77.48 17.99,77.5 | 17.89,77.61 17.99,77.5 | 23.78,88.23 22.13,84.72 22.05,84.67 14.89,84.64 C9.1 | 34.73,88.1 S2.2
  Top 1.27: 34.78,87.95 S2.2 | C7.1 8.62,55.41 C8.1 | S2.2 34.6,88.23 | S2.2 33.61,89.21 29.9,89.21 28.91,88.22 28.91,88.23 J7.1 23.78,88.23
IO-0
  Top 0.381: IC1.30 59.61,73.7 57.41,76.18 38.31,76.18 37.12,74.4 R14.1
IO-1
  Top 0.356: R13.1 40.11,65.74 40.16,65.79 40.16,72.65
  Top 0.381: IC1.31 58.81,64.85 58.78,70.47 58.78,73.01 56.98,75.27 45.19,75.27 43.39,72.83 40.16,72.83 40.16,72.65
IO-2
  Top 0.381: IC1.32 58.01,64.63 57.39,65.26 C18.1
  Top 0.711: R19.2 C18.1
IO-3
  Top 0.381: SW1.D 55.31,71.4 55.48,71.23 55.73,71.23 | 55.73,71.23 R21.2 | IC1.1 55.99,62.09 55.73,62.34 55.73,71.23
L+
  Top 1.27: SV2.3 109.25,23.2 109.3,23.25 109.93,23.89 J4.1 123.05,23.89 D3.A
L-
  Top 1.27: SV2.4 111.84,12.94 111.84,19.44 113.79,21.39 J4.2 125.43,21.39 126.24,22.21 D12.C 127.72,39.45 128.86,40.6 128.86,47.58 126.09,50.35 | C6.P$2 106.92,33.97 106,34.88 106,74.05 109.36,78.42 J5.2 113.54,81.59 120.08,81.59 123.02,78.65 123.02,73.11 126.22,69.91 126.22,51.21 125.91,50.91 125.91,50.53 126.09,50.35 | D10.C 126.09,50.35
L-MIC
  Top 0.305: 57.88,28.43 IC2.13 59.62,28.48 60.41,27.69 60.41,16.29 59.37,15.25 55.18,15.25 54.39,14.46 54.39,9.91 56.01,8.29 58.58,8.29 61.7,11.41 65.03,11.41 X1.2
LEFT-IN
  Top 0.305: SV1.3 45.14,23.81 48.09,20.86 48.09,19.9 48.95,19.03 52.64,19.03 53.78,20.18 53.78,29.37 53.4,29.75 IC2.3
MISO
  Top 0.457: IC1.16 63.61,54.33 64.4,52.33 64.4,46.74 U$4.1
MOSI
  Top 0.457: U$4.4 61.93,41.31 61.93,43.42 60.61,44.69 60.61,48.73 61.8,49.54 62.82,49.54 62.81,53.95 IC1.15
N$1
  Top 0.61: C2.2 45.83,27.97 45.4,28.41 C1.2
N$2
  Top 0.406: IC2.7 C2.1
N$3
  Top 0.381: C3.2 18.07,25.18 18.4,24.85 20.23,24.85 C4.2
N$4
  Top 0.381: IC3.7 23.45,24.67 C4.1
N$5
  Top 1.27: J7.3 26.63,64.27 SW2.2
N$6  (1 unrouted)
  Top 0.889: U1.1 11.94,57.72 | D8.CATHODE 11.92,57.44 12.17,57.18
  Top 1.27: 11.94,57.72 C7.2
N$7
  Top 0.711: 0.44,4.99 0.44,-5.17
N$9
  Top 1.27: D11.A 112.94,44.25 R9.1
N$10
  Top 1.27: D12.A 112.88,39.45 R6.1
N$11
  Top 1.27: D11.C 125.99,44.43 125.99,46.01 124.95,47.05 113.01,47.05 112.53,47.53 D10.A
N$12
  Top 1.27: R1.1 88.68,33.97 D6.C
N$13
  Top 1.27: R2.2 111.11,34.04 | 111.11,34.04 C6.P$1 | 111.11,34.04 111.11,35.97 109.53,37.55 R6.2 109.53,44.31 R9.2 109.56,54.51 R4.3 R4.2
N$14
  Top 1.27: J5.1 117.63,78.42 118.7,77.35 118.7,57.11 R4.1
N$15
  Top 0.889: D1.CATHODE 22.94,69.91 23.88,70.85 23.88,79.46 22.36,80.98 16.54,80.98 15.37,79.81 U2.1 14.64,81.16 C9.2
N$16
  Top 1.27: R1.2 99.52,33.97 C5.P$1 99.68,39.63 R5.2 99.63,45.42 R7.2 99.47,50.6 97.36,52.71 93.05,52.71 92.74,53.02 R3.2 R3.3
N$17
  Top 0.711: -4.64,-0.09 5.52,-0.09
N$18
  Top 1.27: R7.1 93,45.58 D4.A
N$19
  Top 1.27: R5.1 91.14,39.68 D5.A
N$20
  Top 1.27: D4.C 82.73,47.73 82.89,47.89 93.81,47.89 93.81,50.43 90.58,50.43 D2.A
N$21
  Top 1.27: J6.1 90.1,78.11 92.28,78.11 93.55,76.84 93.55,64.4 96.35,61.6 96.35,56.09 R3.1
N$26
  Top 0.381: 46.21,63.99 50.4,63.99 Q1.2 50.4,61.45 51.04,60.82 52.18,60.82 53.32,59.67 53.32,57.77 53.8,57.29 IC1.7
  Top 0.508: C11.1 R11.2 46.21,63.99
N$27
  Top 0.356: Q1.1 50.4,56.37 50.4,56.88 50.79,56.49
  Top 0.381: IC1.8 50.52,56.49 | 50.52,56.49 50.4,56.37 | C12.1 50.22,58.43 50.52,57.52 50.52,56.49
  Top 0.508: R11.1 C12.1
N$28
  Top 0.406: U$2.1 68.43,50.91 R16.1
N$29
  Top 0.889: SW1.B 50.31,87.1 48.88,87.1 48.75,87.23 R18.1
N$30
  Top 0.889: C16.2 M1.6
N$31
  Top 0.406: SW1.A 55.31,83.79 54.92,83.17 43.03,83.14 42.4,82.53 R22.1
  Top 0.889: SW1.A 55.31,88.33 R20.1 R17.1
N$32
  Top 0.889: R20.2 C17.1
N$33  (1 unrouted)
  Top 1.143: D1.ANODE 15.55,64.22 | 15.55,64.22 15.55,62.39 | SW2.1 15.55,64.22
N$34
  Top 0.406: R14.2 33.89,56.8
  Top 0.61: M1.4 15.86,50 16.21,50.35 20.23,50.35 21.95,52.08 23.55,52.08 28.28,56.8 R14.2
N$35
  Top 0.61: M1.5 18.4,47.86 18.37,47.89 19.34,48.85 21.55,48.85 23.04,50.35 24.67,50.35 29.42,55.1 39.61,55.1 40.11,55.61 R13.2
N$36
  Top 0.508: R21.1 60.81,74.74 R15.1
N$37
  Top 0.406: R23.2 42.32,71.41 44,71.38 45.98,74.05 52.94,74.07 52.94,72.32 54.08,71.18 R19.1
N$38
  Top 0.406: R23.1 38.56,73.59 39.5,74.99 R22.2
N$39
  Top 0.889: J15.2 47.23,10.52 46.51,9.81 J1.2
N$40
  Top 0.762: U$4.6 59.34,38.62 60.61,37.35 J14.1
N$41
  Top 0.559: J13.2 50.96,23.1 51.26,23.4 IC2.8
N$42
  Top 0.889: J1.5 34.66,12.32 33.03,13.95 J11.2
N$43
  Top 0.889: SW1.C 52.81,85.48 52.38,85.05 45.65,85.05 44.76,85.94 J17.1
N$44
  Top 0.356: IC3.13 29.95,28.48 29.8,28.33 29.8,22.16 31.3,20.66 31.3,19.44 31.66,19.08 38.87,19.08 39.02,19.24 J16.1
N$45
  Top 0.356: IC2.10 56.83,24.67 55.84,25.66 55.84,33.56 56.37,34.09 56.37,35.72 56.17,35.92 52.13,35.92 51.8,35.59 J21.2
N$46
  Top 0.356: J20.P$2 48.52,36.36 49.16,36.99 57.18,36.99 57.46,36.71 57.46,33.66 56.65,32.85 56.65,26.25 56.95,25.94 IC2.11
N$47
  Top 0.356: IC2.9 56.62,23.4 54.87,25.15 54.87,30.51 54.44,30.95 J19.2
N$48
  Top 0.356: IC2.6 50.96,25.94 50.58,26.32 44.53,26.32 40.57,30.28 J18.2
N$49
  Top 0.305: IC2.15 61.93,31.02 64.47,28.48 J22.1
N$50
  Top 1.27: D3.C 117.28,34.2 R2.1
R+
  Top 1.27: SV2.2 106.71,23.2 106.76,23.25 106.02,23.99 J3.1 D6.A
R-
  Top 1.27: SV2.1 104.17,19.39 104.22,19.44 103.69,21.49 J3.2 85.91,21.49 80.85,26.55 80.85,39.56 | 80.85,39.56 D5.C | 80.85,39.56 79.58,40.83 79.58,49.64 D2.C 80.4,74.1 84.39,78.09 J6.2 87.58,82.55 88.22,83.19 96.09,83.19 102.44,76.34 102.44,34.55 C5.P$2
R-MIC
  Top 0.305: X5.2 81.57,7.45 79.97,5.85 75.57,5.85 73.34,3.61 66.48,3.64 65.26,4.86 59.29,4.83 57.78,3.32 54.93,3.32 53.12,5.14 53.12,9.3
  Top 0.406: 53.12,9 53.12,9.3 53.12,14.26 52.51,14.87 44.66,14.87 43.39,13.6 J16.2
RESET
  Top 0.356: U$4.5 59.34,44.43 60.64,43.14 60.64,39.02 61.14,38.51 62.69,38.51 63.2,39.02 63.2,43.21 63.48,43.49 66.7,43.49 67.62,44.41 67.62,44.53 67.62,44.54 67.62,46.74 69.02,48.32 72.65,48.32 74.38,49.64 74.38,60.26 71.03,63.64 65.03,63.64 64.22,62.82 64.22,62.81 63.62,62.21 60.48,62.21 60.41,62.28 IC1.29 60.41,68.11 62.26,69.96 62.26,75.32 60.51,77.07 40.55,77.07 39.4,77.76 S2.3 S2.4
  Top 0.508: 59.11,46.62 59.04,46.69 57.87,46.69 57.56,46.39 57.56,39.73 57.23,39.4 J9.2
  Top 0.635: 59.11,46.62 U$4.5
RESET1  (1 unrouted)
  Top 0.61: J9.1 25.15,39.4 24.44,38.69 C16.1
  Top 0.66: R12.2 16.75,38.33 D7.ANODE 20.5,38.26
RIGHT-IN
  Top 0.356: IC3.3 27.64,29.75 27.92,29.42 27.92,19.13 28.25,18.73 28.96,18.02 41.1,18.02 SV1.1
S0
  Top 0.356: 43.39,43.44 38.97,43.44 36.33,40.75 36.31,36.99 36.31,31.14 36.3,31.01 36.3,29.37 32.7,25.92 32.67,25.94 IC3.11
  Top 0.406: IC1.11 59.61,52.86 58.2,51.44 55.25,51.44 51.85,48.04 J20.P$1 47.99,48.04 43.39,43.44
S1
  Top 0.356: IC3.10 33.71,24.67 37.75,28.63 37.73,40.65 39.33,42.4 43.11,42.4 43.92,42.4
  Top 0.406: IC1.12 60.41,52.19 58.35,50.12 55.28,50.12 51.52,46.36 J21.1 51.06,42.4 43.11,42.4
S2
  Top 0.356: IC3.9 34.91,23.38 39.1,27.62 39.1,40.39 39.66,41.21 | 55.71,48.29 54.44,47.02 J19.1
  Top 0.406: IC1.13 61.21,51.28 58.93,49 56.42,49 55.71,48.29 | J19.1 54.08,40.32 48.65,40.32 47.76,41.21 39.66,41.21
SCK
  Top 0.356: R16.2 68.24,54.01 66.22,54.01 | IC1.17 65.15,56.45 65.67,56.45 66.22,55.89 66.22,55.66 66.22,55.65 66.22,54.01 | U$4.3 61.88,44.92 62.16,44.64 62.16,44.61 65.87,44.61 66.22,44.96 66.22,54.01
SCL
  Top 0.381: IC1.28 61.21,67.57 63.23,69.58 63.23,74.66 66.15,77.58 JP1.3 R8.1
SDA
  Top 0.381: IC1.27 62.01,66.46 64.37,68.82 64.37,73.77 68.69,78.09 JP1.2 R10.1
VCC  (4 unrouted)
  Top 0.305: IC1.6 57.82,58.09 57.84,58.07
  Top 0.406: IC1.4 56.5,59.67 55.35,59.67 54.97,59.29 54.97,58.28 55.16,58.09 IC1.6
VCC1
  Top 0.406: IC2.16 60.31,32.29 60.59,32.57 60.59,34.65
  Top 0.61: C1.1 45.4,34.32 44.25,35.47 J10.2
  Top 0.762: J10.2 46.08,36.61 46.11,36.58 46.11,37.5 46.79,38.18 57.79,38.18 58.45,37.52 58.45,35.8 59.6,34.65 60.59,34.65 62.97,34.65 63.05,34.58 63.41,34.93
  Top 0.889: U$4.2 64.42,35.95 63.41,34.93 63.41,32.62 64.34,31.68 71.2,31.68 73.15,29.73 J8.2 73.15,20.14 69.3,16.29 69.3,6.59 | 69.3,6.59 70.16,5.72 70.26,5.82 X5.5 | X1.5 56.98,6.59 69.3,6.59
(copper drawn outside any net)
  shapes: Top area x5

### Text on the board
Top: Fab14. Young. Kim / 2018.06.21. R0.1 | Audio Selector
